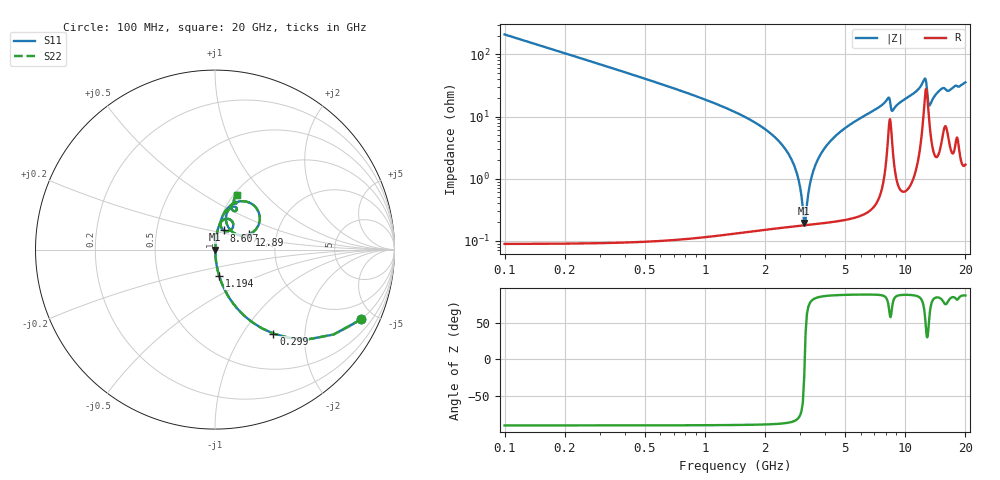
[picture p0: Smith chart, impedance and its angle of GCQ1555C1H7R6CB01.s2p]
!Murata Part Number: GCQ1555C1H7R6CB01
!These Parameters are Measured in Series Mode Connection
!Data Generated on Jan 08, 2026
!  o--ll--o
!Port1  Port2
!  o------o
!Operation Temp=25[degC], DC Bias Voltage=0[V]
!Freq. Start=100[MHz] Stop=20[GHz] 401[Steps]
# Hz S RI R 50
!Freq.(Hz) S11(Real) S11(Imag) S21(Real) S21(Imag) S12(Real) S12(Imag) S22(Real) S22(Imag)
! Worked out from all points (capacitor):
!   401 points, 100 MHz to 20 GHz, reference 50 ohm
!   read as one part in series: C = 7.6 pF near 199.5 MHz
!   lowest |Z| = 194 mohm at 3.135 GHz (marker M1)
!   series resonance near 3.153 GHz, so ESL is about 340 pH
!   S11 on the Smith chart (normalised r, x): 100 MHz: 1.00, -4.18; 299 MHz: 1.00, -1.39; 1.194 GHz: 1.00, -0.30; 8.607 GHz: 1.08, +0.23; 12.89 GHz: 1.44, +0.25; 20 GHz: 1.03, +0.71
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1e8  0.8139 -0.389  0.1861 0.389  0.1861 0.389  0.8139 -0.389
2.99e8  0.3253 -0.4678  0.6747 0.4678  0.6747 0.4678  0.3253 -0.4678
5.975e8  0.1031 -0.3026  0.8969 0.3026  0.8969 0.3026  0.1031 -0.3026
1.1945e9  0.0231 -0.1464  0.9769 0.1464  0.9769 0.1464  0.0231 -0.1464
2.5875e9  0.00235 -0.0263  0.9976 0.0263  0.9976 0.0263  0.00235 -0.0263
2.886e9  0.00186 -0.0118  0.9981 0.0118  0.9981 0.0118  0.00186 -0.0118
3.13475e9  0.00177 -0.000773  0.9982 0.000773  0.9982 0.000773  0.00177 -0.000773
3.23425e9  0.0018 0.00338  0.9982 -0.00338  0.9982 -0.00338  0.0018 0.00338
3.43325e9  0.00196 0.0113  0.998 -0.0113  0.998 -0.0113  0.00196 0.0113
3.7815e9  0.00249 0.0243  0.9975 -0.0243  0.9975 -0.0243  0.00249 0.0243
4.42825e9  0.00417 0.0463  0.9958 -0.0463  0.9958 -0.0463  0.00417 0.0463
6.7665e9  0.0169 0.1162  0.9831 -0.1162  0.9831 -0.1162  0.0169 0.1162
8.20925e9  0.0724 0.1715  0.9276 -0.1715  0.9276 -0.1715  0.0724 0.1715
8.60725e9  0.0502 0.1065  0.9498 -0.1065  0.9498 -0.1065  0.0502 0.1065
1.005e10  0.0417 0.1842  0.9583 -0.1842  0.9583 -0.1842  0.0417 0.1842
1.2438e10  0.2046 0.2551  0.7954 -0.2551  0.7954 -0.2551  0.2046 0.2551
1.288575e10  0.1884 0.0845  0.8116 -0.0845  0.8116 -0.0845  0.1884 0.0845
1.31345e10  0.1022 0.0948  0.8978 -0.0948  0.8978 -0.0948  0.1022 0.0948
1.338325e10  0.0701 0.1323  0.9299 -0.1323  0.9299 -0.1323  0.0701 0.1323
1.497525e10  0.0906 0.2354  0.9094 -0.2354  0.9094 -0.2354  0.0906 0.2354
1.67165e10  0.0922 0.2318  0.9078 -0.2318  0.9078 -0.2318  0.0922 0.2318
2e10  0.1235 0.3061  0.8765 -0.3061  0.8765 -0.3061  0.1235 0.3061
